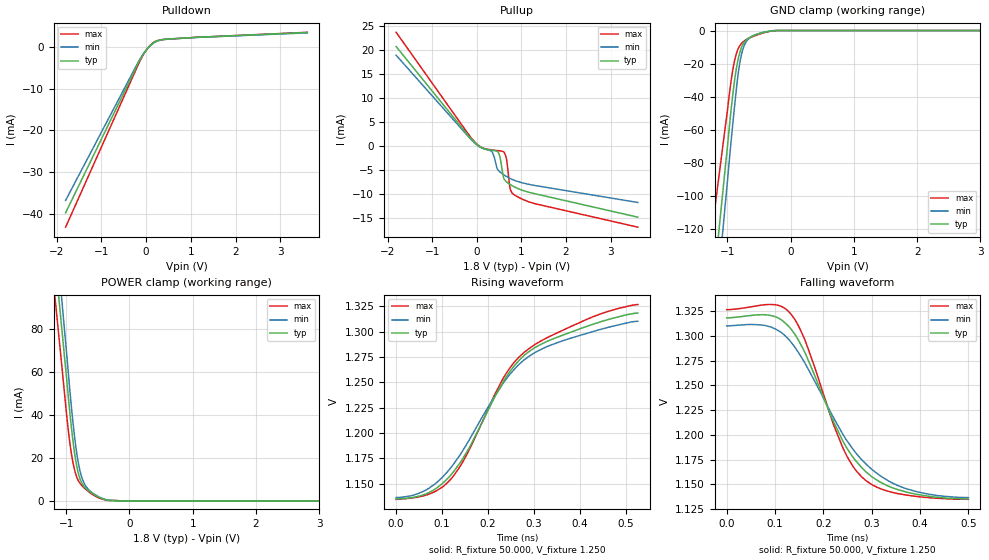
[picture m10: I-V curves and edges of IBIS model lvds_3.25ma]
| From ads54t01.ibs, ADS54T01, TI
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[Model]   lvds_3.25ma
Model_type 3-state
Vref=1.250E+00
Rref=5.000E+01
Cref=0.000E+00
Vmeas=1.250E+00
C_comp   7.860E-13   7.790E-13   7.930E-13
[Voltage Range]   1.800E+00   1.650E+00   1.950E+00
[POWER Clamp Reference]   1.800E+00   1.650E+00   1.950E+00
[GND Clamp Reference]   0.000E+00   0.000E+00   0.000E+00
[Pullup Reference]   1.800E+00   1.650E+00   1.950E+00
[Pulldown Reference]   0.000E+00   0.000E+00   0.000E+00
[Temperature Range]   25   85   -40
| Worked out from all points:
|   slope of the pulldown table from 0 to 0.27 V, typ, clamps not added: 115 ohm
|   slope of the pullup table from 0 to 0.27 V, typ, clamps not added: 244 ohm
|   GND clamp passes 1 mA (typ) near -0.41 V on its own axis
|   POWER clamp passes 1 mA (typ) near -0.41 V on its own axis
|   rising waveform, R_fixture 50.000, V_fixture 1.250: 20-80 % time 153ps typ, 161ps min, 159ps max; typ from 1.14 V to 1.32 V
|   falling waveform, R_fixture 50.000, V_fixture 1.250: 20-80 % time 107ps typ, 128ps min, 87.4ps max; typ from 1.32 V to 1.14 V
[GND Clamp]
-1.8V     -374.4mA   -423.5mA   -288.4mA
-1.02V    -78.69mA   -100.5mA   -54.92mA
-920mV    -41.17mA   -59.34mA   -25.51mA
-860mV    -23.88mA   -36.88mA   -14.48mA
-820mV    -15.94mA   -23.97mA   -10.43mA
-780mV    -10.76mA   -15.27mA   -8.038mA
-740mV    -7.589mA   -9.923mA   -6.562mA
-700mV    -5.657mA   -6.755mA   -5.499mA
-640mV    -4.069mA   -4.329mA   -4.359mA
-460mV    -1.489mA   -1.354mA   -1.806mA
-220mV    -4.201uA   -14.01uA   -11.29uA
3.6V      0A         0A         0A
[Power Clamp]
-1.8V     302.8mA    334.3mA    279.3mA
-1.76V    290.6mA    320.1mA    266.6mA
-1.06V    77.25mA    90.47mA    60.21mA
-940mV    40.5mA     50.88mA    26.54mA
-880mV    24.97mA    33.1mA     16.1mA
-820mV    14.43mA    19.78mA    10.24mA
-780mV    10.23mA    13.83mA    8.195mA
-720mV    6.913mA    8.542mA    6.262mA
-580mV    3.451mA    3.702mA    2.982mA
-360mV    441.4uA    538.8uA    356.5uA
-140mV    0A         9.789uA    18.55uA
3.6V      0A         0A         0A
[Pullup]
-1.81V    20.77mA    18.96mA    23.74mA
-30mV     573.9uA    483.4uA    689.7uA
350mV     -876.7uA   -1.287mA   -813.1uA
470mV     -1.21mA    -4.935mA   -935.5uA
510mV     -1.96mA    -5.329mA   -975.7uA
610mV     -6.869mA   -6.01mA    -1.268mA
670mV     -7.504mA   -6.362mA   -2.981mA
730mV     -7.893mA   -6.67mA    -7.954mA
750mV     -8.01mA    -6.762mA   -9.037mA
790mV     -8.236mA   -6.934mA   -9.798mA
1.29V     -9.903mA   -8.192mA   -11.98mA
3.61V     -14.82mA   -11.75mA   -16.9mA
[Pulldown]
-1.8V     -39.73mA   -36.77mA   -43.18mA
-140mV    -3.143mA   -2.928mA   -3.403mA
-40mV     -1.364mA   -1.295mA   -1.444mA
60mV      1.842uA    -36.81uA   58.98uA
180mV     1.108mA    1.021mA    1.201mA
340mV     1.711mA    1.682mA    1.716mA
540mV     1.917mA    1.921mA    1.887mA
3.6V      3.456mA    3.363mA    3.493mA
[Rising Waveform]
R_fixture = 50.000
V_fixture = 1.250
V_fixture_min = 1.250
V_fixture_max = 1.250
|  time   V(typ)   V(min)   V(max)
0s        1.135V     1.137V     1.135V
66ps      1.14V      1.144V     1.139V
120ps     1.159V     1.167V     1.155V
156ps     1.183V     1.191V     1.181V
232ps     1.25V      1.248V     1.253V
256ps     1.266V     1.262V     1.269V
288ps     1.28V      1.275V     1.283V
338ps     1.292V     1.287V     1.296V
426ps     1.307V     1.3V       1.314V
526ps     1.318V     1.31V      1.327V
[Falling Waveform]
R_fixture = 50.000
V_fixture = 1.250
V_fixture_min = 1.250
V_fixture_max = 1.250
|  time   V(typ)   V(min)   V(max)
0s        1.318V     1.31V      1.327V
88ps      1.321V     1.31V      1.332V
112ps     1.317V     1.304V     1.33V
134ps     1.306V     1.293V     1.321V
164ps     1.281V     1.271V     1.293V
240ps     1.194V     1.201V     1.187V
264ps     1.176V     1.184V     1.166V
288ps     1.163V     1.171V     1.154V
370ps     1.142V     1.146V     1.139V
500ps     1.135V     1.137V     1.135V
[Ramp]
dV/dt_r   1.0980E-01/1.5250E-10   1.0410E-01/1.6090E-10   1.1508E-01/1.5850E-10
dV/dt_f   1.0980E-01/1.0691E-10   1.0410E-01/1.2806E-10   1.1508E-01/8.7078E-11
R_load = 50
